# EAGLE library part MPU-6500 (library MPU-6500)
Accelerometer, Gyroscope, 6 Axis Sensor I²C, SPI Output
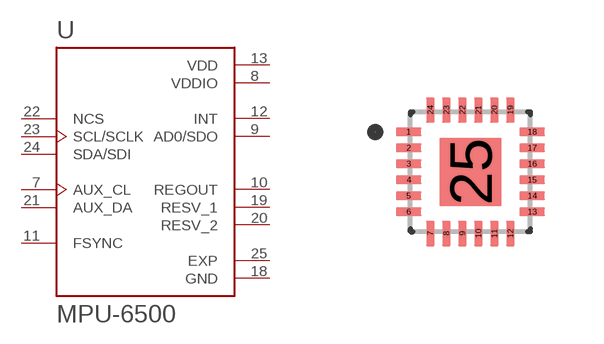
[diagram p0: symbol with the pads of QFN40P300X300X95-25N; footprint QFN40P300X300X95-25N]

Designator prefix U

## MPU-6500 (Check_prices: https://www.snapeda.com/parts/MPU-6500/TDK+InvenSense/view-part/?ref=eda; Description: MotionTracking Device Digital Output 1.8V 24-Pin QFN EP T/R; DigiKey_Part_Number: 1428-1011-2-ND; MF: TDK InvenSense; MP: MPU-6500; Package: QFN-24 TDK; SnapEDA_Link: https://www.snapeda.com/parts/MPU-6500/TDK+InvenSense/view-part/?ref=snap)  [QFN40P300X300X95-25N]
7  AUX_CL  in
8  VDDIO  pwr
9  AD0/SDO  out
10  REGOUT  out
11  FSYNC  in
12  INT  out
13  VDD  pwr
18  GND  pwr
19  RESV_1  pas
20  RESV_2  pas
21  AUX_DA
22  NCS  in
23  SCL/SCLK  in
24  SDA/SDI
25  EXP  pas

## Footprint QFN40P300X300X95-25N (pad centres in mm)
smd 0.64 x 0.22: 1 -1.545,1; 2 -1.545,0.6; 3 -1.545,0.2; 4 -1.545,-0.2; 5 -1.545,-0.6; 6 -1.545,-1; 13 1.545,-1; 14 1.545,-0.6; 15 1.545,-0.2; 16 1.545,0.2; 17 1.545,0.6; 18 1.545,1
smd 0.22 x 0.64: 7 -1,-1.545; 8 -0.6,-1.545; 9 -0.2,-1.545; 10 0.2,-1.545; 11 0.6,-1.545; 12 1,-1.545; 19 1,1.545; 20 0.6,1.545; 21 0.2,1.545; 22 -0.2,1.545; 23 -0.6,1.545; 24 -1,1.545
smd 1.54 x 1.7: 25 0,0

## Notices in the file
This work is licensed under a Creative Commons Attribution-ShareAlike 4.0 International License (CC BY-SA) with Design Exception 1.0
